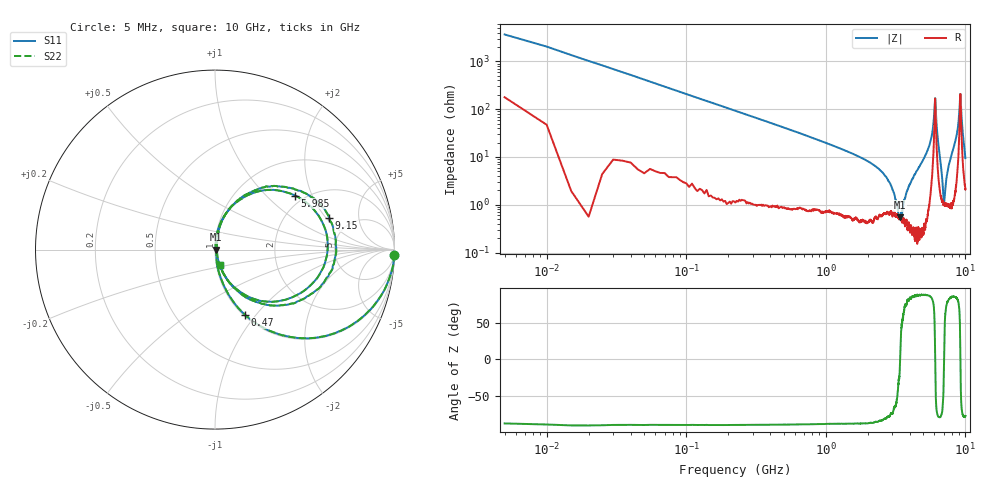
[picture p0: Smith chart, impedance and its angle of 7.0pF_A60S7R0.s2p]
! Amotech Co.,Ltd.
! http://www.amotech.co.kr/
! Part Number: A60S7R0
! These Parameters are Measured in Series Mode Connection
! Operation Temp=25[degC], DC Bias Voltage=0[V]
! Freq. Start=5[MHz] Stop=10[GHz], 2000[Steps]
! Date: Monday, July 13, 2020, 01:32:05
# GHZ S RI R 50.000000
!Freq.(Hz) S11(Real) S11(Imag) S21(Real) S21(Imag) S12(Real) S12(Imag) S22(Real) S22(Imag)
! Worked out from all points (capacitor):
!   2000 points, 5 MHz to 10 GHz, reference 50 ohm
!   read as one part in series: C = 7.68 pF near 55 MHz
!   lowest |Z| = 551 mohm at 3.4 GHz (marker M1)
!   series resonance near 3.404 GHz, so ESL is about 280 pH
!   S11 on the Smith chart (normalised r, x): 5 MHz: 5, -73; 470 MHz: 1.02, -0.88; 5.985 GHz: 1.79, +1.51; 9.15 GHz: 3.45, +2.16; 10 GHz: 1.04, -0.18
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0.005  0.9979 -0.0273  0.00208 0.0273  0.00208 0.0273  0.9979 -0.0273
0.07  0.8942 -0.2999  0.1058 0.2999  0.1058 0.2999  0.8942 -0.2999
0.13  0.715 -0.4451  0.285 0.4451  0.285 0.4451  0.715 -0.4451
0.47  0.1669 -0.3629  0.8331 0.3629  0.8331 0.3629  0.1669 -0.3629
1.675  0.0161 -0.1037  0.9839 0.1037  0.9839 0.1037  0.0161 -0.1037
2.73  0.00796 -0.0358  0.992 0.0358  0.992 0.0358  0.00796 -0.0358
3.34  0.00535 -0.00252  0.9946 0.00252  0.9946 0.00252  0.00535 -0.00252
3.4  0.00546 -0.000558  0.9945 0.000558  0.9945 0.000558  0.00546 -0.000558
3.955  0.00434 0.0248  0.9957 -0.0248  0.9957 -0.0248  0.00434 0.0248
5.005  0.0104 0.0886  0.9896 -0.0886  0.9896 -0.0886  0.0104 0.0886
5.73  0.0898 0.2378  0.9102 -0.2378  0.9102 -0.2378  0.0898 0.2378
5.985  0.4459 0.3009  0.5541 -0.3009  0.5541 -0.3009  0.4459 0.3009
6.075  0.6269 -0.00727  0.3731 0.00727  0.3731 0.00727  0.6269 -0.00727
6.185  0.3334 -0.2895  0.6666 0.2895  0.6666 0.2895  0.3334 -0.2895
6.67  0.0189 -0.0643  0.9811 0.0643  0.9811 0.0643  0.0189 -0.0643
7.035  0.0107 0.000164  0.9893 -0.000164  0.9893 -0.000164  0.0107 0.000164
7.455  0.0122 0.0493  0.9878 -0.0493  0.9878 -0.0493  0.0122 0.0493
8.335  0.0429 0.1682  0.9571 -0.1682  0.9571 -0.1682  0.0429 0.1682
8.835  0.1827 0.311  0.8173 -0.311  0.8173 -0.311  0.1827 0.311
9.15  0.6365 0.1767  0.3635 -0.1767  0.3635 -0.1767  0.6365 0.1767
9.385  0.3787 -0.3099  0.6213 0.3099  0.6213 0.3099  0.3787 -0.3099
10  0.0287 -0.0876  0.9713 0.0876  0.9713 0.0876  0.0287 -0.0876
